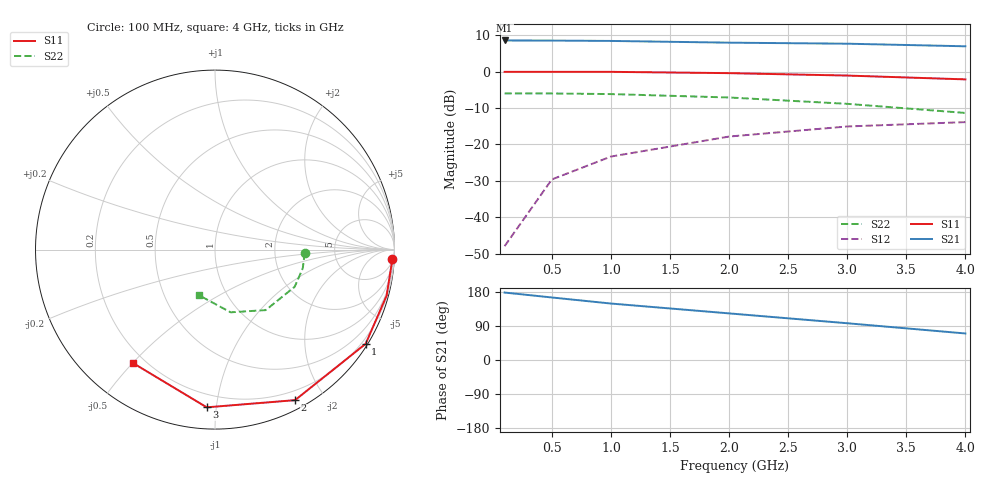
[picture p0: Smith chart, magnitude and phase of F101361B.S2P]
!ATF-10136
!S-PARAMETERS at Vds=1V  Id=5mA.  LAST UPDATED 06-29-94
# ghz s ma r 50
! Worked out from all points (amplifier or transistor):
!   6 points, 100 MHz to 4 GHz, reference 50 ohm
!   highest |S21| = 8.5 dB at 100 MHz (marker M1)
!   |S21| within 3 dB of that: start of sweep to end of sweep
!   unconditionally stable (mu >= 1): nowhere
!   at 500 MHz: K = 0.15, MSG = 19.1 dB, |S12| = -29.6 dB
!   at 2 GHz: K = 0.22, MSG = 12.9 dB, |S12| = -17.9 dB
!   at 4 GHz: K = 0.49, MSG = 10.4 dB, |S12| = -13.9 dB
!   lowest NFmin = 0.40 dB at 500 MHz
!   S11 on the Smith chart (normalised r, x): 100 MHz: 7, -37; 1 GHz: 0.07, -3.49; 2 GHz: 0.10, -1.66; 3 GHz: 0.12, -0.94; 4 GHz: 0.16, -0.50
0.1  0.99 -3.0  2.67 178.0  0.004 98.0  0.5 -2.0
0.5  0.99 -15.0  2.66 165.0  0.033 76.0  0.5 -12.0
1  0.99 -32.0  2.63 149.0  0.068 68.0  0.49 -25.0
2  0.95 -62.0  2.49 123.0  0.128 44.0  0.44 -50.0
3  0.88 -93.0  2.41 97.0  0.176 29.0  0.36 -76.0
4  0.78 -126.0  2.22 70.0  0.202 7.0  0.27 -109.0
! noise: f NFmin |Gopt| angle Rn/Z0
0.5  0.4  0.93  12  0.85
1  0.4  0.85  24  0.7
2  0.4  0.7  47  0.46
4  0.5  0.39  126  0.36
